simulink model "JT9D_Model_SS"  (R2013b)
settings: Solver=FixedStepDiscrete  StartTime=0.0  StopTime=10.0  FixedStep=0.2  RelTol=1e-3
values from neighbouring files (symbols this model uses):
  MWS = setup_Inputs(MWS)    [JT9D_setup_everything_Dyn.m]    (also in JT9D_setup_everything_SS.m; Tsetup_Ambient.m = MWS; GasTurbine_Dyn_setup_everything.m = setup_Duct(MWS))
libraries: Lib_Turbo_Duct_TMATS x5, Lib_Turbo_Compressor_TMATS x3, Lib_Turbo_Shaft_TMATS x2, Lib_Turbo_TurbineNPSS_TMATS x2, Lib_Turbo_Nozzle_TMATS x2, Lib_Turbo_Burner_TMATS x1, Lib_Turbo_Inlet_TMATS x1, Lib_Turbo_Splitter_TMATS x1, Lib_Solve_SSNRSolverJC_TMATS x1

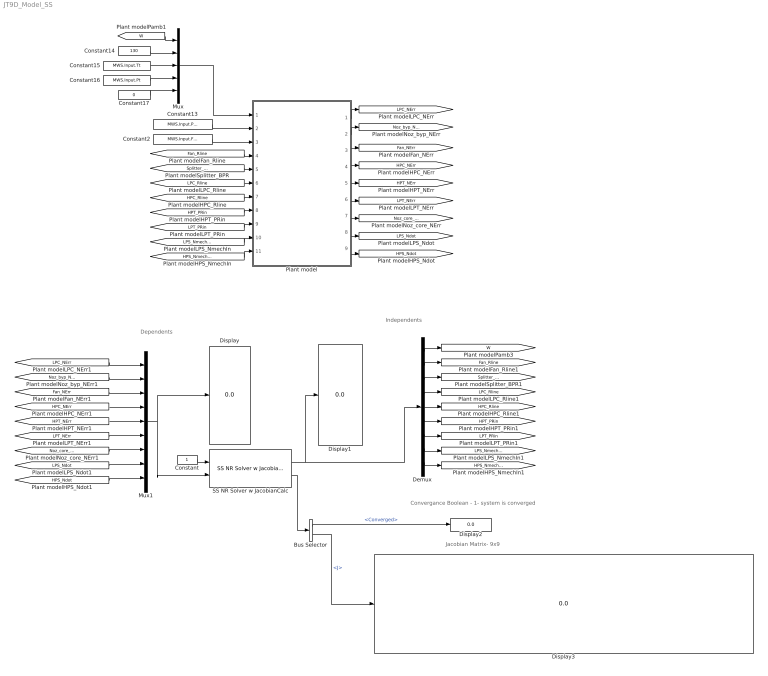
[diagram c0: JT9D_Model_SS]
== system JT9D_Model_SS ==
  note: Jacobian Matrix- 9x9
  note: Dependents
  note: Independents
  note: Convergance Boolean - 1- system is converged
  Bus Selector : BusSelector  OutputSignals=Converged,J
  Constant : Constant
  Constant13 : Constant  Value=MWS.Input.Pamb
  Constant14 : Constant  Value=130
  Constant15 : Constant  Value=MWS.Input.Tt
  Constant16 : Constant  Value=MWS.Input.Pt
  Constant17 : Constant  Value=0
  Constant2 : Constant  Value=MWS.Input.FARin
  Demux : Demux  Outputs=9
  Display{,1..3} (4 alike) : Display
  Mux : Mux  Inputs=5
  Mux1 : Mux  Inputs=9
  Plant model : Subsystem
  SS NR Solver w JacobianCalc : Lib_Solve_SSNRSolverJC_TMATS/SS NR Solver w JacobianCalc  SJac_Per_M=[0.05 0.05 0.05 0.05 0.05 0.05 0.05 0.05 0.05 ]  SNR_IC_M=MWS.Input.NRIC  SNR_DX_M=1  SJacobianAttempts_M=20  Cond_Limits_M=0.005
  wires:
  Mux/1 -> Plant model/1(Input GPC)
  Constant17/1 -> Mux/5
  Constant15/1 -> Mux/3
  Constant16/1 -> Mux/4
  Constant14/1 -> Mux/2
  Constant13/1 -> Plant model/2(Pamb)
  Constant2/1 -> Plant model/3(FAR_dmd)
  [Fan_Rline] -> Plant model/4(Fan_Rline)
  [Splitter_BPR] -> Plant model/5(Splitter_BPR)
  [LPC_Rline] -> Plant model/6(LPC_Rline)
  [HPC_Rline] -> Plant model/7(HPC_Rline)
  [HPT_PRin] -> Plant model/8(HPT_PRin)
  [LPT_PRin] -> Plant model/9(LPT_PRin)
  [LPS_NmechIn] -> Plant model/10(LPS_NmechIn)
  [HPS_NmechIn] -> Plant model/11(HPS_NmechIn)
  Plant model/1(LPC_NErr) -> [LPC_NErr]
  Plant model/2(Noz_byp_NErr) -> [Noz_byp_NErr]
  Plant model/3(Fan_NErr) -> [Fan_NErr]
  Plant model/4(HPC_NErr) -> [HPC_NErr]
  Plant model/5(HPT_NErr) -> [HPT_NErr]
  Plant model/6(LPT_NErr) -> [LPT_NErr]
  Plant model/7(Noz_core_NErr) -> [Noz_core_NErr]
  Plant model/8(LPS_Ndot) -> [LPS_Ndot]
  Plant model/9(HPS_Ndot) -> [HPS_Ndot]
  [W] -> Mux/1
  Demux/1 -> [W]
  Demux/7 -> [LPT_PRin]
  Demux/5 -> [HPC_Rline]
  Demux/6 -> [HPT_PRin]
  Demux/4 -> [LPC_Rline]
  Demux/8 -> [LPS_NmechIn]
  Demux/9 -> [HPS_NmechIn]
  Demux/2 -> [Fan_Rline]
  Demux/3 -> [Splitter_BPR]
  [Fan_NErr] -> Mux1/3
  [HPC_NErr] -> Mux1/4
  [Noz_byp_NErr] -> Mux1/2
  [HPT_NErr] -> Mux1/5
  [LPC_NErr] -> Mux1/1
  [LPT_NErr] -> Mux1/6
  [Noz_core_NErr] -> Mux1/7
  SS NR Solver w JacobianCalc/2 -> Bus Selector/1
  Mux1/1 -> SS NR Solver w JacobianCalc/2, Display/1
  Bus Selector/1 -> Display2/1  "<Converged>"
  Bus Selector/2 -> Display3/1  "<J>"
  [LPS_Ndot] -> Mux1/8
  [HPS_Ndot] -> Mux1/9
  SS NR Solver w JacobianCalc/1 -> Demux/1, Display1/1
  Constant/1 -> SS NR Solver w JacobianCalc/1

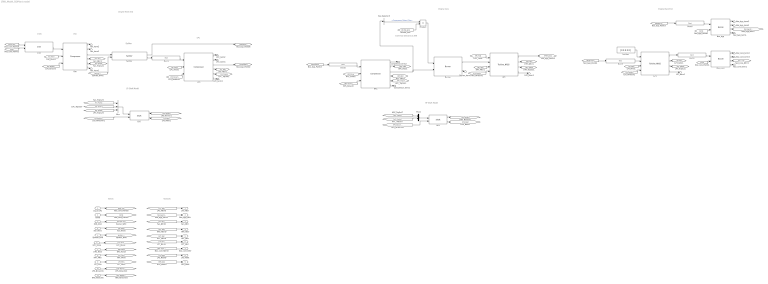
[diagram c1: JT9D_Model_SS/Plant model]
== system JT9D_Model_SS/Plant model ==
  note: LP Shaft Model
  note: Inputs
  note: Outputs
  note: Engine Core
  note: HP Shaft Model
  note: Engine Back End
  note: Engine Front End
  note: Fuel Flow demand as FAR
  note: Inlet
  note: Fan
  note: Splitter
  note: LPC
  Input GPC : Inport
  Pamb : Inport  Port=2
  FAR_dmd : Inport  Port=3
  Fan_Rline : Inport  Port=4
  Splitter_BPR : Inport  Port=5
  LPC_Rline : Inport  Port=6
  HPC_Rline : Inport  Port=7
  HPT_PRin : Inport  Port=8
  LPT_PRin : Inport  Port=9
  LPS_NmechIn : Inport  Port=10
  HPS_NmechIn : Inport  Port=11
  Burner : Lib_Turbo_Burner_TMATS/Burner  LHV_M=18400  dPnormBurner_M=MWS.Burn.dP  Eff_M=0.994
  Burner_term1 : Terminator
  Bus Selector5 : BusSelector  OutputSignals=Compressor Output Flow; WOut[pps]
  Compressor_term1 : Terminator
  Compressor_term2 : Terminator
  Duct1 : Lib_Turbo_Duct_TMATS/Duct  dP_M=MWS.Duct.dP1
  Duct2 : Lib_Turbo_Duct_TMATS/Duct  dP_M=MWS.Duct.dP2
  Duct3 : Lib_Turbo_Duct_TMATS/Duct  dP_M=MWS.Duct.dP3
  Duct4 : Lib_Turbo_Duct_TMATS/Duct  dP_M=MWS.Duct.dP4
  Duct5 : Lib_Turbo_Duct_TMATS/Duct  dP_M=MWS.Duct.dP5
  Fan : Lib_Turbo_Compressor_TMATS/Compressor  X_C_RlineVec_M=MWS.FAN.RlineVec  Y_C_NcVec_M=MWS.FAN.NcVec  T_C_Map_WcArray_M=MWS.FAN.WcArray  T_C_Map_PRArray_M=MWS.FAN.PRArray  T_C_Map_EffArray_M=MWS.FAN.EffArray  s_C_Nc_M=MWS.FAN.s_Nc  s_C_Wc_M=MWS.FAN.s_Wc  s_C_PR_M=MWS.FAN.s_PR  s_C_Eff_M=MWS.FAN.s_eff  CBLDEN_M=off  C_CBD_M=0  C_CBFht_M=0.5  C_CBFPt_M=0.5  FBLDEN_M=off  C_FBD_M=0  C_BFht_M=0.5  C_BFPt_M=0.5  X_C_WcSurgeVec_M=[0 5000]  T_C_PRSurgeVec_M=[30 30]  iDesign_M=MWS.iDes  NcDes_M=1  EffDes_M=0.8675  PRDes_M=1.645  RlineDes_M=2.3706  FVar_M='iDesScalars.mat'  SVar_M=gcb  NcNm_M='_C_Nc'  WcNm_M='_C_Wc'  PRNm_M='_C_PR'  EffNm_M='_C_Eff'
  Fan_term1 : Terminator
  Fan_term2 : Terminator
  Fan_term3 : Terminator
  HPC : Lib_Turbo_Compressor_TMATS/Compressor  X_C_RlineVec_M=MWS.HPC.RlineVec  Y_C_NcVec_M=MWS.HPC.NcVec  T_C_Map_WcArray_M=MWS.HPC.WcArray  T_C_Map_PRArray_M=MWS.HPC.PRArray  T_C_Map_EffArray_M=MWS.HPC.EffArray  s_C_Nc_M=MWS.HPC.s_Nc  s_C_Wc_M=MWS.HPC.s_Wc  s_C_PR_M=MWS.HPC.s_PR  s_C_Eff_M=MWS.HPC.s_eff  CBLDEN_M=off  C_CBD_M=0  C_CBFht_M=0.5  C_CBFPt_M=0.5  FBLDEN_M=on  C_FBD_M=MWS.HPC.Fbld  C_BFht_M=MWS.HPC.Fblde  C_BFPt_M=MWS.HPC.Fbldp  X_C_WcSurgeVec_M=[0 200]  T_C_PRSurgeVec_M=[30 30]  iDesign_M=MWS.iDes  NcDes_M=0.995  EffDes_M=.8651  PRDes_M=5.609  RlineDes_M=2.0424  FVar_M='iDesScalars.mat'  SVar_M=gcb  NcNm_M='_C_Nc'  WcNm_M='_C_Wc'  PRNm_M='_C_PR'  EffNm_M='_C_Eff'
  HPS : Lib_Turbo_Shaft_TMATS/Shaft  Shaft_Inertia_M=1000
  HPT : Lib_Turbo_TurbineNPSS_TMATS/Turbine_NPSS  X_T_PRVec_M=MWS.HPT.PRVec  Y_T_NcVec_M=MWS.HPT.NcVec  T_T_Map_WcArray_M=MWS.HPT.WcArray  T_T_Map_EffArray_M=MWS.HPT.EffArray  s_T_Nc_M=MWS.HPT.s_Nc  s_T_Wc_M=MWS.HPT.s_Wc  s_T_PR_M=MWS.HPT.s_PR  s_T_Eff_M=MWS.HPT.s_eff  CFlwEn_M=on  T_CoolFlwPos_M=MWS.HPT.Cool  iDesign_M=MWS.iDes  NcDes_M=99.031  EffDes_M=.9133  PRDes_M=4.930  NDes_M=7390  FVar_M='iDesScalars.mat'  SVar_M=gcb  NcNm_M='_C_Nc'  WcNm_M='_C_Wc'  PRNm_M='_C_PR'  EffNm_M='_C_Eff'
  HPT_term1 : Terminator
  Inlet : Lib_Turbo_Inlet_TMATS/Inlet  eRambase_M=MWS.Inlet.eRamBase  X_eRamVec_M=MWS.Inlet.eRamVec  T_eRamtbl_M=MWS.Inlet.eRamtbl
  LPC : Lib_Turbo_Compressor_TMATS/Compressor  X_C_RlineVec_M=MWS.LPC.RlineVec  Y_C_NcVec_M=MWS.LPC.NcVec  T_C_Map_WcArray_M=MWS.LPC.WcArray  T_C_Map_PRArray_M=MWS.LPC.PRArray  T_C_Map_EffArray_M=MWS.LPC.EffArray  s_C_Nc_M=MWS.LPC.s_Nc  s_C_Wc_M=MWS.LPC.s_Wc  s_C_PR_M=MWS.LPC.s_PR  s_C_Eff_M=MWS.LPC.s_eff  CBLDEN_M=off  C_CBD_M=0  C_CBFht_M=0.5  C_CBFPt_M=0.5  FBLDEN_M=off  C_FBD_M=0  C_BFht_M=0.5  C_BFPt_M=0.5  X_C_WcSurgeVec_M=[0 200]  T_C_PRSurgeVec_M=[30 30]  iDesign_M=MWS.iDes  NcDes_M=0.993  EffDes_M=.8683  PRDes_M=2.488  RlineDes_M=1.7664  FVar_M='iDesScalars.mat'  SVar_M=gcb  NcNm_M='_C_Nc'  WcNm_M='_C_Wc'  PRNm_M='_C_PR'  EffNm_M='_C_Eff'
  LPC_term1 : Terminator
  LPC_term2 : Terminator
  LPC_term3 : Terminator
  LPS : Lib_Turbo_Shaft_TMATS/Shaft  Shaft_Inertia_M=1000
  LPT : Lib_Turbo_TurbineNPSS_TMATS/Turbine_NPSS  X_T_PRVec_M=MWS.LPT.PRVec  Y_T_NcVec_M=MWS.LPT.NcVec  T_T_Map_WcArray_M=MWS.LPT.WcArray  T_T_Map_EffArray_M=MWS.LPT.EffArray  s_T_Nc_M=MWS.LPT.s_Nc  s_T_Wc_M=MWS.LPT.s_Wc  s_T_PR_M=MWS.LPT.s_PR  s_T_Eff_M=MWS.LPT.s_eff  CFlwEn_M=off  T_CoolFlwPos_M=0  iDesign_M=MWS.iDes  NcDes_M=105.038  EffDes_M=.9323  PRDes_M=6.420  NDes_M=3667.6  FVar_M='iDesScalars.mat'  SVar_M=gcb  NcNm_M='_C_Nc'  WcNm_M='_C_Wc'  PRNm_M='_C_PR'  EffNm_M='_C_Eff'
  LPT_term1 : Terminator
  Mux : Mux  Inputs=3
  Mux1 : Mux  Inputs=2
  NoFlow : Constant  Value=[0 0 0 0 0]
  Noz_byp : Lib_Turbo_Nozzle_TMATS/Nozzle  SWType_M=1  N_TArea_M=MWS.NozB.Ath  N_EArea_M=110.7  N_FL_M=0.00  X_N_TtVec2_M=[300 2000]  T_N_TGArray_M=[1 1]  X_N_PEQPaVec_M=[0 10000]  T_N_CdThArray_M=[1 1]  T_N_CvArray_M=MWS.NozB.CvArray  T_N_CfgArray_M=[1 1]  X_N_FARVec_M=[0; 0.0050; 0.0100; 0.0150; 0.0200; 0.0250; 0.0300]  T_N_RtArray_M="[0.0686;    0.0686;    0.0686;    0.0686;    0.0686;    0.0686;    0.0686]"  Y_N_TtVec_M=[300 2000]  T_N_MAP_gammaArray_M=[ 1.4 1.4 1.4 1.4 1.4 1.4 1.4; 1.4 1.4 1.4 1.4 1.4 1.4 1.4]  iDesign_M=MWS.iDes  WDes_M=562.61  FVar_M='iDesScalars.mat'  SVar_M=gcb  AthNm_M='_Ath'  AxNm_M='_Ax'
  Noz_byp_term1 : Terminator
  Noz_byp_term2 : Terminator
  Noz_byp_term3 : Terminator
  Noz_core : Lib_Turbo_Nozzle_TMATS/Nozzle  SWType_M=1  N_TArea_M=MWS.Noz.Ath  N_EArea_M=110.7  N_FL_M=0.00  X_N_TtVec2_M=[300 2000]  T_N_TGArray_M=[1 1]  X_N_PEQPaVec_M=[0 10000]  T_N_CdThArray_M=[1 1]  T_N_CvArray_M=MWS.Noz.CvArray  T_N_CfgArray_M=[1 1]  X_N_FARVec_M=[0; 0.0050; 0.0100; 0.0150; 0.0200; 0.0250; 0.0300]  T_N_RtArray_M="[0.0686;    0.0686;    0.0686;    0.0686;    0.0686;    0.0686;    0.0686]"  Y_N_TtVec_M=[300 2000]  T_N_MAP_gammaArray_M=[ 1.4 1.4 1.4 1.4 1.4 1.4 1.4; 1.4 1.4 1.4 1.4 1.4 1.4 1.4]  iDesign_M=MWS.iDes  WDes_M=113.51  FVar_M='iDesScalars.mat'  SVar_M=gcb  AthNm_M='_Ath'  AxNm_M='_Ax'
  Noz_core_term1 : Terminator
  Noz_core_term2 : Terminator
  Noz_core_term3 : Terminator
  Product : Product
  Splitter : Lib_Turbo_Splitter_TMATS/Splitter
  LPC_NErr : Outport
  Noz_byp_NErr : Outport  Port=2
  Fan_NErr : Outport  Port=3
  HPC_NErr : Outport  Port=4
  HPT_NErr : Outport  Port=5
  LPT_NErr : Outport  Port=6
  Noz_core_NErr : Outport  Port=7
  LPS_Ndot : Outport  Port=8
  HPS_Ndot : Outport  Port=9
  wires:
  Fan_Rline/1 -> [Fan_Rline]
  HPS_NmechIn/1 -> [HPS_NmechIn]
  HPC_Rline/1 -> [HPC_Rline]
  LPT_PRin/1 -> [LPT_PRin]
  FAR_dmd/1 -> [Wf_FAR_dmd]
  Splitter_BPR/1 -> [Splitter_BPR]
  LPC_Rline/1 -> [LPC_Rline]
  HPT_PRin/1 -> [HPT_PRin]
  LPS_NmechIn/1 -> [LPS_NmechIn]
  Duct1/1 -> LPC/1
  Duct4/1 -> Noz_core/1
  HPC/6 -> Compressor_term1/1
  Noz_core/4 -> Noz_core_term1/1
  [Pamb] -> Noz_core/2
  Noz_core/3 -> [Noz_core_NErr]
  Duct3/1 -> LPT/2
  Noz_core/2 -> Noz_core_term3/1
  Mux/1 -> LPS/1
  Mux1/1 -> HPS/1
  [LPT_TrqOut] -> Mux/3
  [Fan_TrqOut] -> Mux/1
  [HPT_TrqOut] -> Mux1/2
  [HPC_TrqOut] -> Mux1/1
  [LPC_TrqOut] -> Mux/2
  HPS/2 -> [HPS_Ndot]
  HPS/1 -> [HPS_Nmech]
  [LPS_Nmech] -> Fan/3
  [LPS_Nmech] -> LPT/4
  [HPS_NmechIn] -> HPS/2
  [HPS_Nmech] -> HPC/3
  [LPS_Nmech] -> LPC/3
  Duct2/1 -> HPC/1
  Duct5/1 -> Noz_byp/1
  LPT/2 -> [LPT_NErr]
  [LPT_PRin] -> LPT/3
  LPT/4 -> LPT_term1/1
  [HPS_Nmech] -> HPT/4
  LPS/2 -> [LPS_Ndot]
  LPS/1 -> [LPS_Nmech]
  [LPS_NmechIn] -> LPS/2
  HPT/4 -> HPT_term1/1
  Splitter/2 -> Duct1/1
  Fan/3 -> Splitter/1
  Splitter/1 -> [BypassFlowOut]
  Burner/1 -> HPT/2
  LPT/1 -> Duct4/1
  LPC/3 -> [LPCFlowOut]
  HPT/2 -> [HPT_NErr]
  [HPT_PRin] -> HPT/3
  NoFlow/1 -> LPT/1
  Inlet/1 -> Fan/1
  LPT/3 -> [LPT_TrqOut]
  HPC/1 -> Compressor_term2/1
  Noz_byp/3 -> [Noz_byp_NErr]
  [Fan_Rline] -> Fan/2
  Noz_byp/1 -> Noz_byp_term3/1
  HPT/3 -> [HPT_TrqOut]
  Noz_byp/4 -> Noz_byp_term1/1
  [Pamb] -> Noz_byp/2
  Noz_byp/2 -> Noz_byp_term2/1
  Burner/2 -> Burner_term1/1
  LPC/2 -> LPC_term3/1
  LPC/4 -> [LPC_NErr]
  LPC/1 -> LPC_term2/1
  LPC/5 -> [LPC_TrqOut]
  [LPC_Rline] -> LPC/2
  [Splitter_BPR] -> Splitter/2
  [HPC_Fbld] -> HPT/1
  Fan/5 -> [Fan_TrqOut]
  Fan/4 -> [Fan_NErr]
  Fan/2 -> Fan_term3/1
  Fan/6 -> Fan_term1/1
  Fan/1 -> Fan_term2/1
  HPC/5 -> [HPC_TrqOut]
  [HPC_Rline] -> HPC/2
  HPC/4 -> [HPC_NErr]
  HPC/2 -> [HPC_Fbld]
  LPC/6 -> LPC_term1/1
  [LPC_NErr] -> LPC_NErr/1
  [Noz_byp_NErr] -> Noz_byp_NErr/1
  [Fan_NErr] -> Fan_NErr/1
  [HPC_NErr] -> HPC_NErr/1
  [HPT_NErr] -> HPT_NErr/1
  [LPT_NErr] -> LPT_NErr/1
  [Noz_core_NErr] -> Noz_core_NErr/1
  [LPS_Ndot] -> LPS_Ndot/1
  [HPS_Ndot] -> HPS_Ndot/1
  [HPTFlowOut] -> Duct3/1
  [Wf_FAR_dmd] -> Product/2
  Bus Selector5/1 -> Product/1  "<Compressor Output Flow; WOut[pps]>"
  Product/1 -> Burner/1
  Pamb/1 -> [Pamb]
  [Pamb] -> Inlet/2
  [Input_GPC] -> Inlet/1
  Input GPC/1 -> [Input_GPC]
  Noz_core/1 -> Noz_core_term2/1
  [LPCFlowOut] -> Duct2/1
  HPT/1 -> [HPTFlowOut]
  [BypassFlowOut] -> Duct5/1
  HPC/3 -> Bus Selector5/1, Burner/2
